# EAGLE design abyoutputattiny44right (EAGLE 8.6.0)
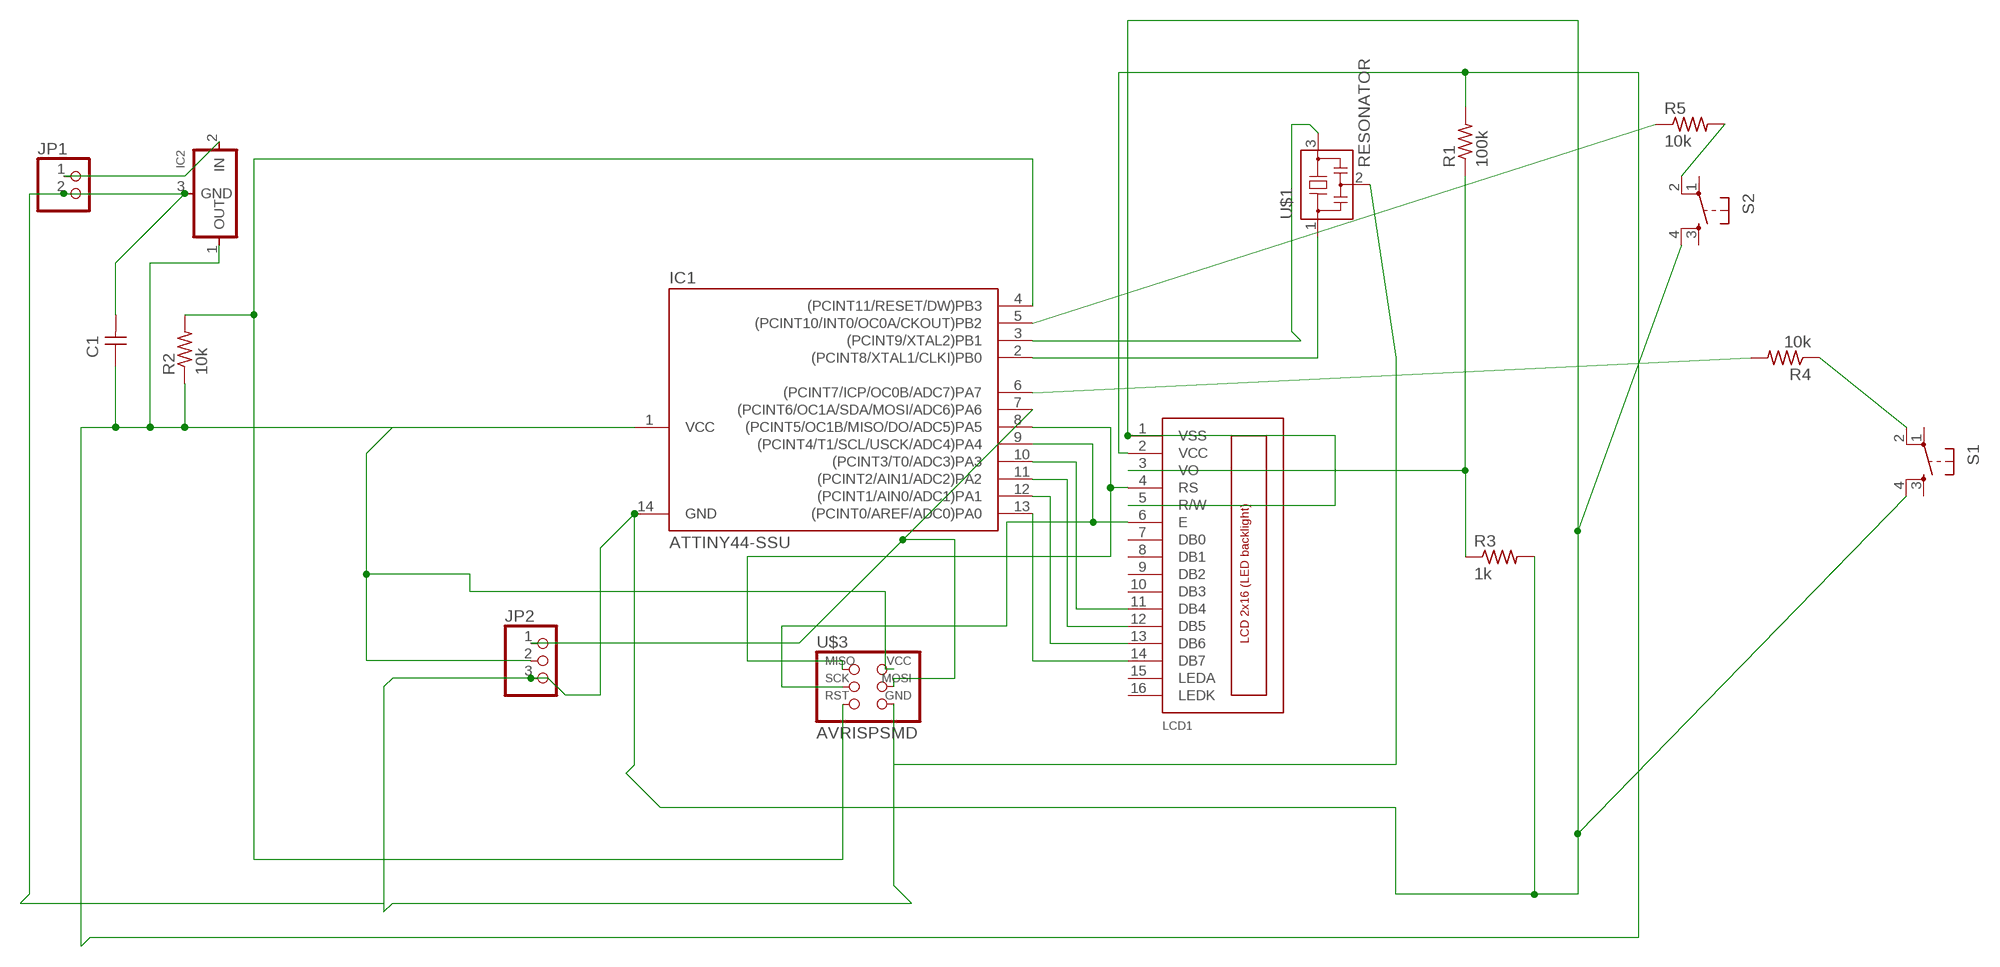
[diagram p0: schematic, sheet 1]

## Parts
C1  CAP-UNPOLARIZEDFAB  [C1206FAB]
IC1  ATTINY44-SSU  [SOIC14]
IC2  REGULATORSOT23  [SOT23]
JP1  PINHD-1X2  [1X02]
JP2  PINHD-1X3  [1X03]
LCD1  LCD_2X16_SIL  [HY-1602F]
R1  100k  RES-US1206FAB  [R1206FAB]
R2  10k  RES-US1206FAB  [R1206FAB]
R3  1k  RES-US1206FAB  [R1206FAB]
R4  10k  RES-US1206FAB  [R1206FAB]
R5  10k  RES-US1206FAB  [R1206FAB]
S1  6MM_SWITCH6MM_SWITCH  [6MM_SWITCH]
S2  6MM_SWITCH6MM_SWITCH  [6MM_SWITCH]
U$1  RESONATOR  [EFOBM]
U$3  AVRISPSMD  [2X03SMD]

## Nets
N$1: IC1.2((PCINT8/XTAL1/CLKI)PB0) U$1.1
N$2: IC1.3((PCINT9/XTAL2)PB1) U$1.3
N$3: U$1.2 U$3.6(GND)
N$4: IC1.4((PCINT11/RESET/DW)PB3) R2.2 U$3.5(RST)
N$5: IC1.13((PCINT0/AREF/ADC0)PA0) LCD1.14(DB7)
N$6: IC1.12((PCINT1/AIN0/ADC1)PA1) LCD1.13(DB6)
N$7: IC1.11((PCINT2/AIN1/ADC2)PA2) LCD1.12(DB5)
N$8: IC1.10((PCINT3/T0/ADC3)PA3) LCD1.11(DB4)
N$9: IC1.9((PCINT4/T1/SCL/USCK/ADC4)PA4) LCD1.6(E) U$3.3(SCK)
N$10: IC1.8((PCINT5/OC1B/MISO/DO/ADC5)PA5) LCD1.4(RS) U$3.1(MISO)
N$11: IC1.7((PCINT6/OC1A/SDA/MOSI/ADC6)PA6) JP2.1 U$3.4(MOSI)
N$12: IC1.14(GND) JP2.3 LCD1.1(VSS) LCD1.5(R/W) R3.2 S1.4(S1) S2.4(S1)
N$14: C1.2 IC2.3(GND) JP1.2
N$15: LCD1.3(VO) R1.1 R3.1
N$16: IC2.2(IN) JP1.1
N$17: IC1.6((PCINT7/ICP/OC0B/ADC7)PA7) R4.2
N$18: R4.1 S1.2(P1)
N$19: IC1.5((PCINT10/INT0/OC0A/CKOUT)PB2) R5.1
N$20: R5.2 S2.2(P1)
N$21: C1.1 IC1.1(VCC) IC2.1(OUT) JP2.2 LCD1.2(VCC) R1.2 R2.1 U$3.2(VCC)
Unconnected: LCD1.7(DB0) LCD1.8(DB1) LCD1.9(DB2) LCD1.10(DB3) LCD1.15(LEDA) LCD1.16(LEDK) S1.1(P) S1.3(S) S2.1(P) S2.3(S)

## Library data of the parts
C1 = fab:CAP-UNPOLARIZED
IC1 = fab:ATTINY44
IC2 = fab:REGULATOR
JP1 = pinhead:PINHD-1X2: PIN HEADER
JP2 = pinhead:PINHD-1X3: PIN HEADER
LCD1 = lcd_2x16_led_backlight:LCD_2X16_SIL
R1-R5 = fab:RES-US: Resistor (US Symbol)
S1 S2 = fab:6MM_SWITCH: OMRON SWITCH
U$1 = fab:RESONATOR
U$3 = fab:AVRISP

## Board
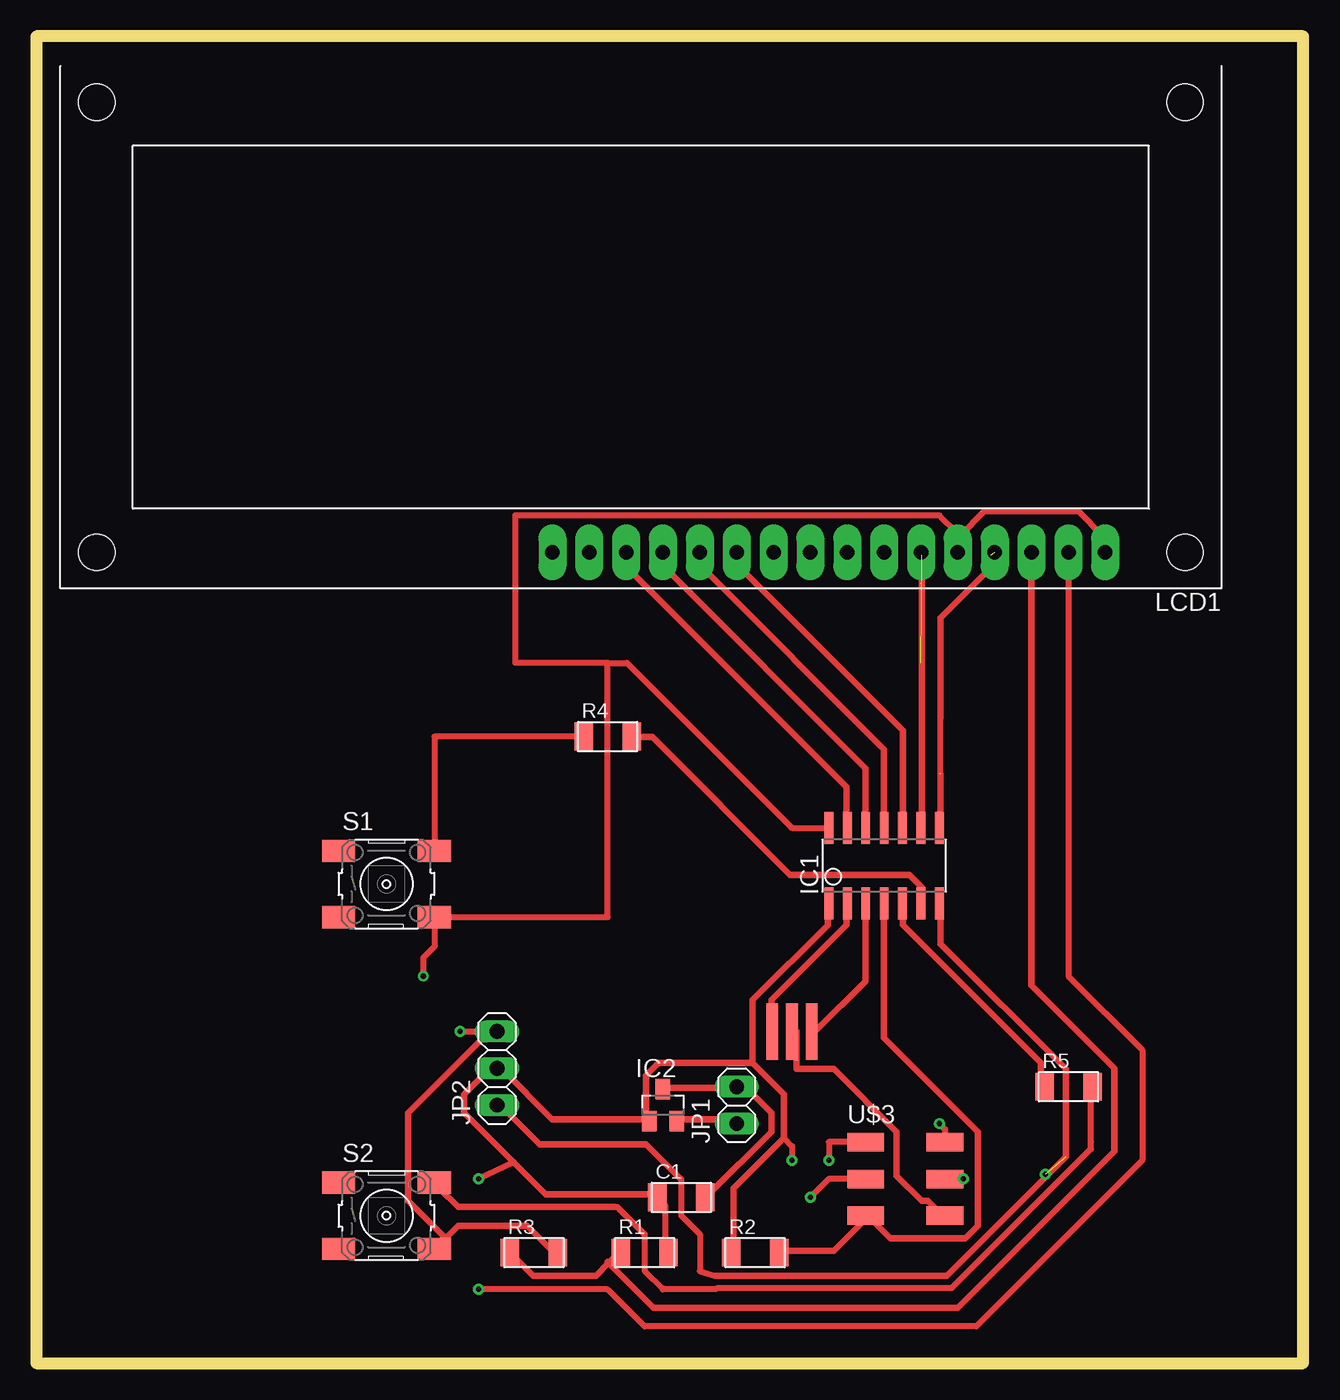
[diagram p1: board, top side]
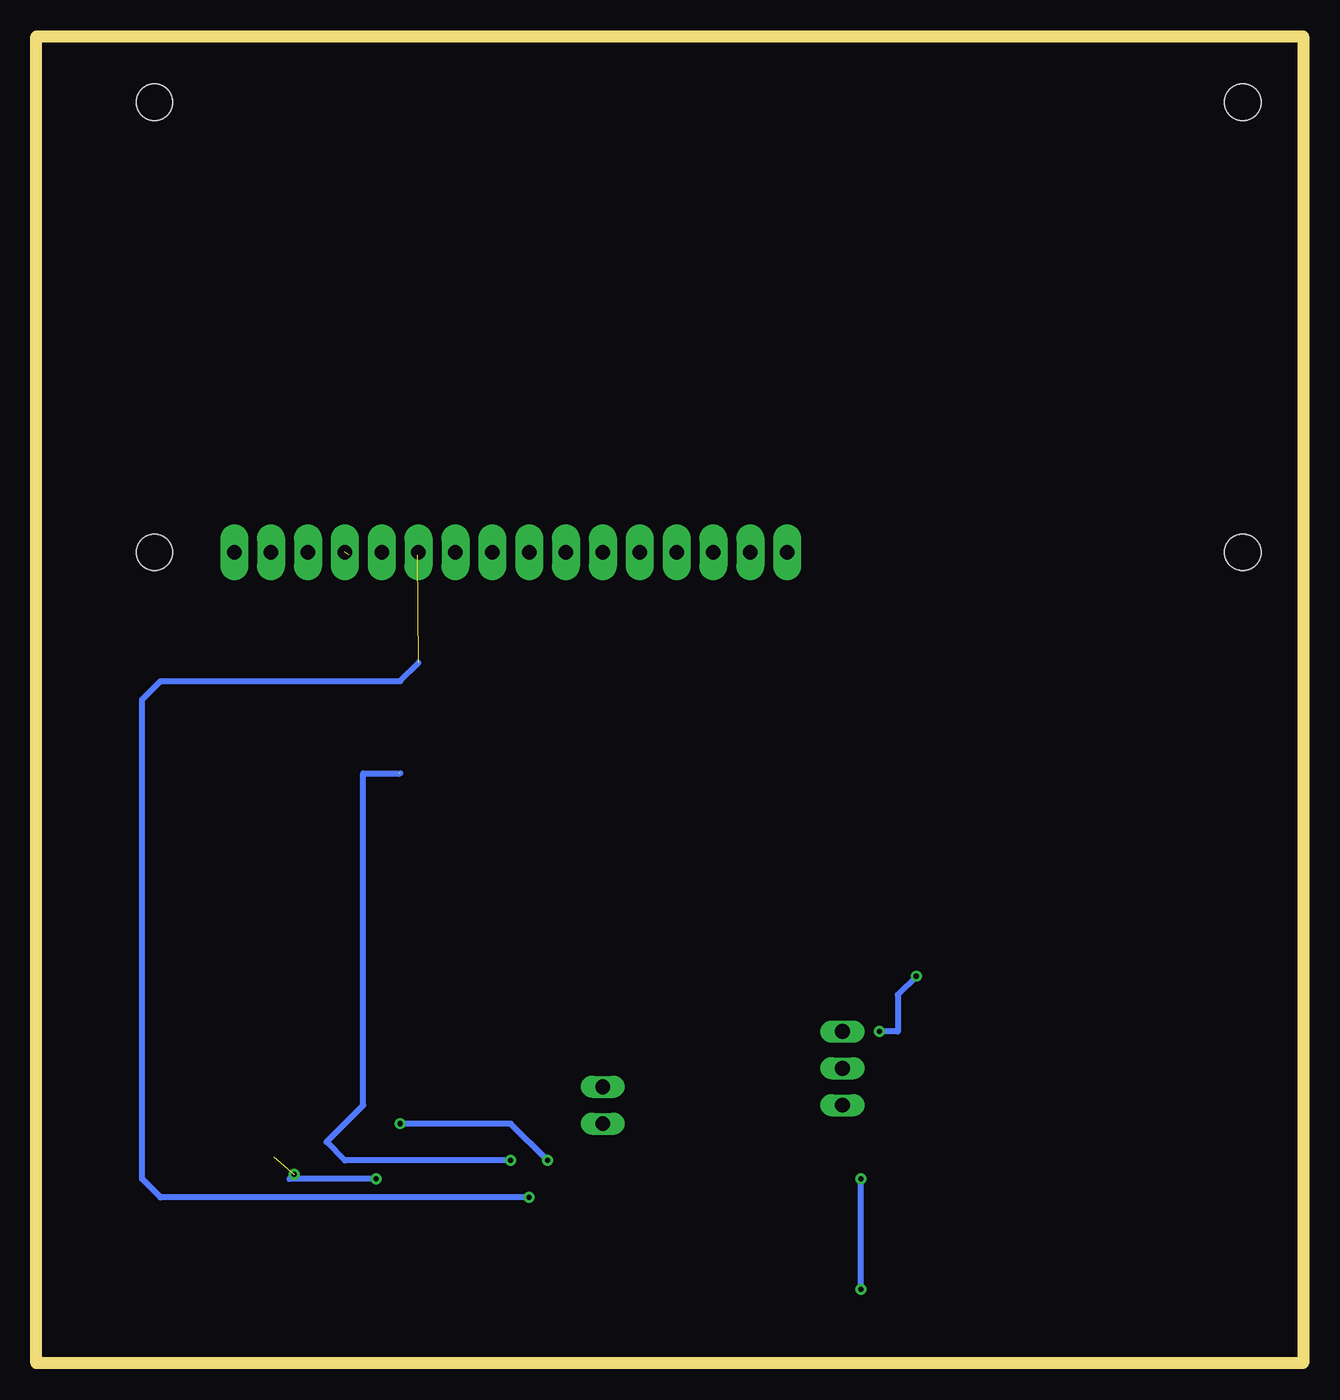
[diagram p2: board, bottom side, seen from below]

Size 87.3 x 91.43 mm. Coordinates in mm from the lower left corner, seen from the top.
Outline: 0,0 87.3,0 87.3,91.43 0,91.43 0,0
Copper layers (1*16): Top 0.035mm / dielectric 1.5mm / Bottom 0.035mm
Design rules "default *": minimum track width 18mil, minimum drill 0.35mm, track to track 16mil, track to pad 16mil, pad to pad 16mil, via to via 16mil, smd to smd 16mil, copper to edge 40mil, drill to drill 6mil, minimum pad ring 10mil, minimum via ring 8mil, stop-mask expansion 4mil, vias tented up to drill 0mil, thermal gap 10mil

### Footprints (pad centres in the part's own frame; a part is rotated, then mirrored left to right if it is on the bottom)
C1206FAB = smd 1.27 x 1.905: 1 -1.651,0; 2 1.651,0
SOIC14 = smd 0.61 x 2.21: 1 -3.81,-2.603; 2 -2.54,-2.603; 3 -1.27,-2.603; 4 0,-2.603; 5 1.27,-2.603; 6 2.54,-2.603; 7 3.81,-2.603; 8 3.81,2.603; 9 2.54,2.603; 10 1.27,2.603; 11 0,2.603; 12 -1.27,2.603; 13 -2.54,2.603; 14 -3.81,2.603
SOT23 = smd 1 x 1.4: 1 -0.95,-1.1; 2 0.95,-1.1; 3 0,1.1
1X02 = drill 1.016 long: 1 -1.27,0; 2 1.27,0
1X03 = drill 1.016 long: 1 -2.54,0; 2 0,0; 3 2.54,0
HY-1602F = drill 1 pad 1.93 long: 1 2.54,0; 2 5.08,0; 3 7.62,0; 4 10.16,0; 5 12.7,0; 6 15.24,0; 7 17.78,0; 8 20.32,0; 9 22.86,0; 10 25.4,0; 11 27.94,0; 12 30.48,0; 13 33.02,0; 14 35.56,0; 15 38.1,0; 16 40.64,0 | hole 2.5: -2.96,0; 72.04,0; -2.96,-31; 72.04,-31
R1206FAB = smd 1.27 x 1.905: 1 -1.651,0; 2 1.651,0
6MM_SWITCH = smd 2.286 x 1.524: 1 -3.302,2.286; 2 3.302,2.286; 3 -3.302,-2.286; 4 3.302,-2.286
EFOBM = smd 0.8 x 3.9: 1 -1.35,0; 2 0,0; 3 1.35,0
2X03SMD = smd 2.54 x 1.27: 1 -2.54,2.54; 2 2.92,2.54; 3 -2.54,0; 4 2.92,0; 5 -2.54,-2.54; 6 2.92,-2.54

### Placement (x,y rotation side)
C1  44.45,11.43 0 top
IC1  58.42,34.29 0 top
IC2  43.18,17.78 0 top
JP1  48.26,17.78 90 top
JP2  31.75,20.32 90 top
LCD1  76.2,55.88 180 top
R1  41.91,7.62 0 top
R2  49.53,7.62 0 top
R3  34.29,7.62 0 top
R4  39.37,43.18 0 top
R5  71.12,19.05 0 top
S1  24.13,33.02 0 top
S2  24.13,10.16 0 top
U$1  52.07,22.86 0 top
U$3  59.69,12.7 0 top

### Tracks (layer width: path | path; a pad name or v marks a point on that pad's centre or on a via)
N$1
  Top 0.457: IC1.2 55.83,31.5 55.83,30.2 50.65,25.02 50.65,22.86 U$1.1
N$2
  Top 0.457: IC1.3 57.12,31.5 57.12,26.31 53.67,22.86 U$1.3
N$3
  Top 0.457: U$3.6 62.31,10.34 61.44,11.2 61.01,11.2 59.28,12.93 59.28,15.95 54.97,20.27 52.38,20.27 52.38,22.86 U$1.2
N$4
  Top 0.457: R2.2 51.51,7.75 54.97,7.75 57.12,9.91 U$3.5 57.56,9.91 58.85,8.61 64.03,8.61 64.9,9.47 64.9,15.95 58.42,22.43 IC1.4
N$5
  Top 0.457: IC1.13 55.83,37.11 55.83,39.7 40.72,54.81 40.72,55.68 LCD1.14
N$6
  Top 0.457: IC1.12 57.12,37.11 57.12,41 43.31,54.81 43.31,55.68 LCD1.13
N$7
  Top 0.457: IC1.11 58.42,42.29 45.9,54.81 45.9,55.68 LCD1.12
N$8
  Top 0.457: IC1.10 59.72,37.11 59.72,43.59 48.49,54.81 48.49,55.68 LCD1.11
N$9  (via drill 0.35)  (1 unrouted)
  Top 0.406: U$3.3 54.61,12.7 v53.34,11.43
  Top 0.457: IC1.9 61.01,37.11 61.01,55.68 LCD1.6
  Bottom 0.406: v53.34,11.43 78.74,11.43 80.01,12.7 80.01,45.72 78.74,46.99 62.23,46.99 60.96,48.26
N$10  (via drill 0.35)  (2 unrouted)
  Top 0.406: U$3.1 54.61,15.24 v54.61,13.97 | 62.31,40.64 62.31,44.45
  Top 0.457: 62.31,44.45 62.31,51.36 65.76,54.81 65.76,55.68 | 62.31,40.64 62.31,37.11 IC1.8
  Bottom 0.406: v54.61,13.97 66.04,13.97 67.31,15.24 64.77,17.78 64.77,40.64 62.23,40.64
N$11  (via drill 0.35)  (1 unrouted)
  Top 0.406: 42.01,15.09 44.4,12.7 44.45,12.7 44.45,10.16 45.72,8.89 45.72,6.35 46.76,6.02 | U$3.4 v63.88,12.7
  Top 0.457: 46.76,6.02 62.74,6.02 70.94,14.22 70.94,20.27 62.31,28.91 62.31,31.5 IC1.7 | 42.01,15.09 34.67,15.09 32.08,17.68 JP2.1
  Bottom 0.406: v63.88,12.7 69.85,12.7 v69.53,13.02
N$12  (via drill 0.35)
  Top 0.406: 52.07,36.89 52.01,36.89 | 63.6,56.97 63.5,56.87 LCD1.5 63.5,57.15 62.23,58.42 33.02,58.42 33.02,48.26 39.37,48.26 | 52.07,36.89 40.7,48.26 39.37,48.26 | 39.37,48.26 39.37,30.73 S1.4 27.43,28.7 26.67,27.94 v26.67,26.67 | 52.07,36.89 IC1.14 | v29.21,22.86 JP2.3
  Top 0.457: 63.6,56.97 65.33,58.7 71.81,58.7 73.53,56.97 73.53,56.11 LCD1.1 | 28.19,8.61 27.76,8.18 S2.4 28.19,8.61 | 28.19,8.61 29.06,9.47 33.81,9.47 35.54,7.75 R3.2 | 54.53,37.11 IC1.14 | 31.65,23.29 31.65,22.86 JP2.3 31.65,23.29 | 28.19,8.61 25.6,11.2 25.6,17.25 31.65,23.29
  Bottom 0.406: v26.67,26.67 27.94,25.4 27.94,22.86 v29.21,22.86
N$14
  Top 0.457: IC2.3 43.31,18.97 48.06,18.97 JP1.2 48.49,19.41 50.65,17.25 50.65,15.95 46.33,11.63 C1.2
N$15
  Top 0.457: R3.1 34.24,6.02 38.56,6.02 39.45,6.91 | 39.45,6.91 39.85,7.31 R1.1 | 68.78,55.68 LCD1.3 68.58,26.04 74.3,20.32 74.3,14.61 63.5,3.81 42.55,3.81 39.45,6.91 | 39.37,6.98 39.45,6.91
N$16
  Top 0.457: IC2.2 44.17,16.82 48.06,16.82 JP1.1
N$17
  Top 0.457: R4.2 41.15,43.16 42.44,43.16 51.94,33.66 60.15,33.66 61.01,32.79 61.01,31.93 IC1.6
N$18
  Top 0.406: R4.1 27.43,43.18 S1.2
  Top 0.457: 37.69,43.16 R4.1
N$19
  Top 0.457: R5.1 69.22,19.41 69.22,20.7 59.72,30.2 59.72,31.5 IC1.5
N$20
  Top 0.406: 39.37,10.77 40.03,10.77 41.91,8.89 41.91,6.35 43.18,5.08 43.24,5.14 46.87,5.14 46.91,5.18 63.09,5.18 72.67,14.77 72.67,15.24 72.67,18.97
  Top 0.457: 39.85,10.77 39.37,10.77 29.06,10.77 27.76,12.06 S2.2 | 72.67,18.97 R5.2
N$21  (via drill 0.35)
  Top 0.406: LCD1.2 71.12,26.67 76.2,21.59 76.2,13.97 64.77,2.54 41.91,2.54 39.37,5.08 v30.48,5.08 | v30.48,12.7 32.89,13.84 | C1.1 43.31,10.92 43.31,7.75 | 51.51,15.52 52.07,14.96 v52.07,13.97 | v62.23,16.51 62.61,16.13 U$3.2
  Top 0.457: 43.31,7.75 R1.2 | 42.01,16.82 35.54,16.82 32.08,20.27 JP2.2 31.65,20.7 29.49,18.54 29.49,17.25 32.89,13.84 35.1,11.63 42.44,11.63 C1.1 | 49.35,20.7 51.51,18.54 51.51,15.52 48.06,12.06 48.06,7.75 R2.1 | 49.35,20.7 42.88,20.7 42.01,19.84 42.01,16.82 | 42.01,16.82 IC2.1 | 49.35,20.7 49.35,25.02 54.53,30.2 54.53,31.5 IC1.1
  Bottom 0.406: v30.48,5.08 v30.48,12.7 | v52.07,13.97 54.61,16.51 v62.23,16.51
